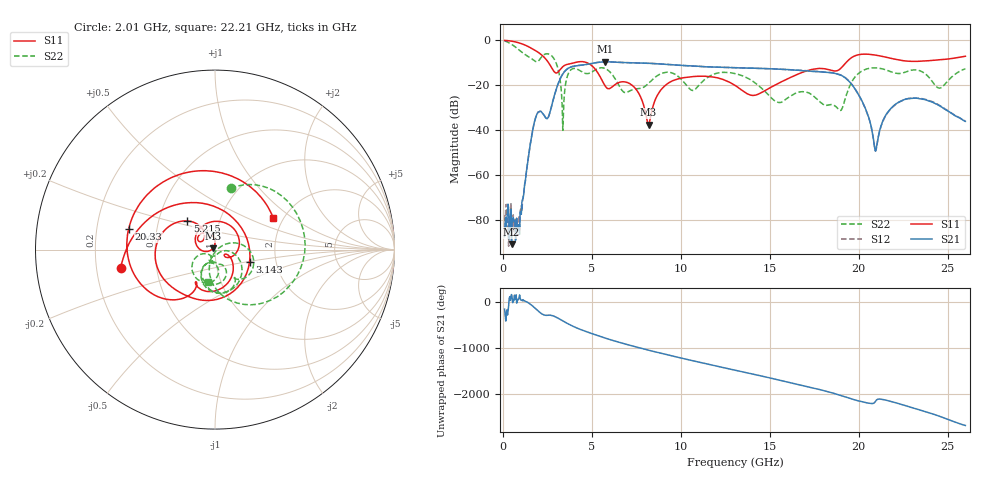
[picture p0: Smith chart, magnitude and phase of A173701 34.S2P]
!  2-Port S-parameters saved by WinCal
! VAR MeasName=S-Parameters (CALIBRATED_DATA) read from VNA (N5245A)
! VAR MeasDate=2017-6-7 10:30:43
! VAR NAME=A173701 34
! VAR FILENAME=A173701 34.S2P
! VAR DATE=2017-6-7 10:30:43
! VAR PHYS_PORTS=1,2
# Hz S DB R 50
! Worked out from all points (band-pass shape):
!   801 points, 100 MHz to 26 GHz, reference 50 ohm
!   highest |S21| = -9.55 dB at 5.733 GHz (marker M1); lowest = -90.9 dB at 488.5 MHz (marker M2)
!   |S21| within 3 dB of the highest: 3.653 GHz to 14.72 GHz (11.07 GHz wide, 120 % of centre)
!   lowest |S11| = -37.6 dB at 8.194 GHz (marker M3), VSWR 1.03, Z = 48.9 + j0.718 ohm
!   |S11| at or under -10 dB: 2.575 GHz to 3.997 GHz (1.422 GHz wide, 43.3 % of centre); 4.745 GHz to 19.28 GHz (14.53 GHz wide, 121 % of centre)
!   |S22| runs from -40.1 to -0.2 dB; largest |S21 - S12| = 0.0042
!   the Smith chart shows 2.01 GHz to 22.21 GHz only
!   S11 on the Smith chart (normalised r, x): 2.01 GHz: 0.31, -0.09; 3.143 GHz: 1.46, -0.22; 5.215 GHz: 0.70, +0.24; 20.33 GHz: 0.34, +0.10; 22.21 GHz: 1.77, +0.73
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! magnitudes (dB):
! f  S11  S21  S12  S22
! 100 MHz  0.0  -87.5  -78.0  -0.2
! 488.5 MHz  -0.3  -90.9  -84.2  -1.7
! 974.1 MHz  -1.3  -76.6  -76.1  -4.6
! 2.01 GHz  -5.4  -31.8  -31.8  -9.1
! 2.528 GHz  -9.5  -34.6  -34.6  -6.0
! 3.143 GHz  -13.8  -18.6  -18.6  -14.1
! 3.402 GHz  -11.5  -14.6  -14.6  -33.2
! 3.758 GHz  -10.4  -12.1  -12.1  -13.7
! 4.438 GHz  -9.4  -11.0  -11.0  -14.0
! 5.215 GHz  -13.1  -10.0  -10.0  -13.0
! 5.733 GHz  -20.1  -9.5  -9.6  -12.5
! 7.255 GHz  -19.9  -10.0  -10.0  -22.1
! 8.194 GHz  -37.6  -10.2  -10.2  -19.1
! 8.744 GHz  -23.7  -10.4  -10.4  -15.4
! 13.05 GHz  -20.0  -12.2  -12.2  -14.8
! 17.39 GHz  -12.9  -13.8  -13.7  -24.4
! 18.97 GHz  -12.6  -15.4  -15.4  -31.2
! 20.33 GHz  -6.1  -29.5  -29.7  -13.1
! 20.95 GHz  -6.6  -49.4  -49.4  -12.2
! 21.69 GHz  -7.8  -31.4  -31.6  -13.6
! 22.21 GHz  -8.6  -27.7  -27.8  -14.8
! 26 GHz  -7.1  -36.1  -36.0  -12.6
